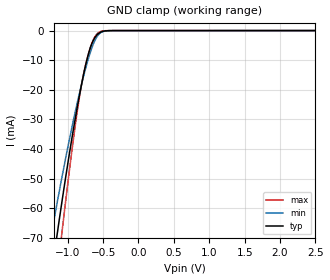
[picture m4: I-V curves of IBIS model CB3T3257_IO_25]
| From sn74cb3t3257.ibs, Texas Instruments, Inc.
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[Model]   CB3T3257_IO_25
Model_type  Terminator
| variable   typ   min   max
C_comp   3.99pF   3.08pF   5.16pF
| C_tri-state   3.99pF   3.08pF   5.16pF
[Temperature Range]   40   100   -40
| Ambient temperature   25   85   -40
[Voltage range]   2.5   2.3   2.7
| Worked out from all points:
|   GND clamp passes 1 mA (typ) near -0.57 V on its own axis
[GND Clamp]
| CB3T3257_IO_25
|   Voltage   I(typ)   I(min)   I(max)
-5.5V     -1.008A    -841.1mA   -1.184A
-1.235V   -83.3mA    -69.49mA   -101mA
-1.19V    -75.63mA   -63.49mA   -91.19mA
-1.145V   -68.12mA   -57.61mA   -81.54mA
-1.08V    -57.57mA   -49.36mA   -67.95mA
-900mV    -30.64mA   -28.16mA   -33.26mA
-795mV    -17.08mA   -17.26mA   -16.99mA
-740mV    -11.03mA   -12.18mA   -10.83mA
-675mV    -5.462mA   -6.985mA   -5.356mA
-565mV    -993.4uA   -1.388mA   -699.2uA
-350mV    -4.598uA   -7.852uA   -524nA
2.5V      184.6pA    1.99nA     62.59pA
